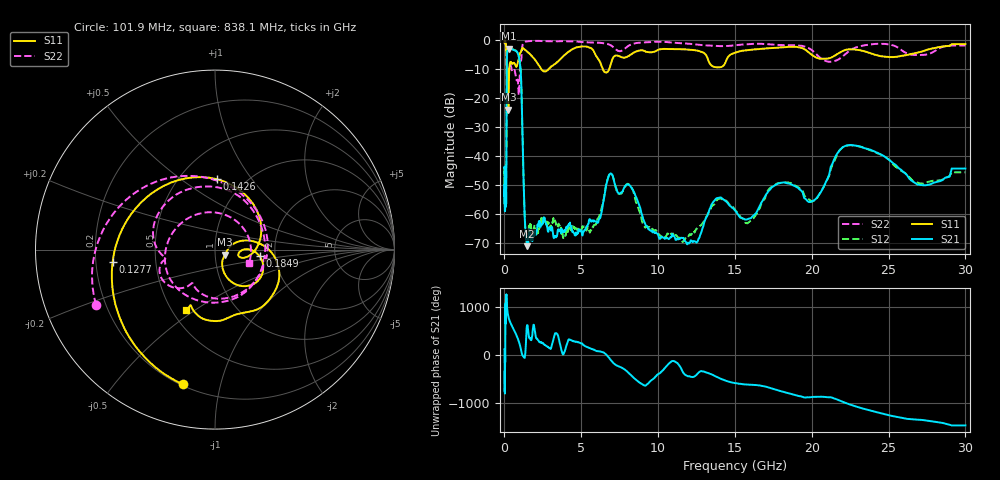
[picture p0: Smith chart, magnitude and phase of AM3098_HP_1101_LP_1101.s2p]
! Date/Time: Thu, Feb 28, 2019 8:46 AM
! Network Analyzer: Agilent Technologies E8364B Rev: A.07.50.67
! Sweep from 0.010 to 30.000 GHz, 1601 Points, Sweep Type: LOG
! Power Supply: 5.022 V, 0.002 A
# Hz S DB R 50
!freq MagS11 AngS11 MagS21 AngS21 MagS12 AngS12 MagS22 AngS22
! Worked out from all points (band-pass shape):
!   1601 points, 10 MHz to 30 GHz, reference 50 ohm
!   highest |S21| = -3.12 dB at 266.5 MHz (marker M1); lowest = -71.2 dB at 1.475 GHz (marker M2)
!   |S21| within 3 dB of the highest: 159.3 MHz to 944.9 MHz (785.6 MHz wide, 142 % of centre)
!   lowest |S11| = -24.1 dB at 252.2 MHz (marker M3), VSWR 1.13, Z = 55.8 - j3.15 ohm
!   |S11| at or under -10 dB: 148 MHz to 316 MHz (168 MHz wide, 72.4 % of centre); 2.372 GHz to 2.902 GHz (529.7 MHz wide, 20.1 % of centre); 6.381 GHz to 6.833 GHz (452.4 MHz wide, 6.85 % of centre)
!   |S22| runs from -19.1 to -0.4 dB; largest |S21 - S12| = 0.012
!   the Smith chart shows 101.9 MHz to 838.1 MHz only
!   S11 on the Smith chart (normalised r, x): 101.9 MHz: 0.21, -0.77; 127.7 MHz: 0.27, -0.06; 142.6 MHz: 0.75, +0.69; 184.9 MHz: 1.65, -0.13; 838.1 MHz: 0.59, -0.46
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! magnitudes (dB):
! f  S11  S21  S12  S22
! 10 MHz  -0.3  -44.3  -44.4  -0.6
! 38.04 MHz  -0.3  -58.3  -58.8  -0.9
! 101.9 MHz  -2.3  -55.3  -56.4  -2.7
! 127.7 MHz  -4.8  -41.3  -41.2  -6.2
! 142.6 MHz  -8.1  -16.8  -16.8  -10.7
! 144.7 MHz  -8.8  -14.3  -14.3  -10.9
! 184.9 MHz  -12.0  -4.1  -4.1  -10.4
! 252.2 MHz  -24.1  -3.2  -3.1  -11.0
! 266.5 MHz  -19.8  -3.1  -3.1  -10.9
! 550.5 MHz  -8.2  -3.5  -3.4  -10.8
! 838.1 MHz  -8.5  -4.4  -4.4  -13.8
! 1.066 GHz  -4.3  -11.4  -11.4  -7.9
! 1.321 GHz  -3.5  -61.6  -61.9  -0.8
! 1.475 GHz  -4.1  -71.2  -69.3  -0.6
! 2.084 GHz  -7.6  -66.5  -66.3  -0.5
! 5.528 GHz  -2.7  -61.9  -66.0  -1.0
! 7.926 GHz  -6.1  -50.1  -50.0  -2.7
! 12.19 GHz  -3.6  -69.4  -67.0  -1.5
! 13.88 GHz  -9.6  -54.6  -55.1  -2.2
! 20.2 GHz  -5.9  -55.2  -55.3  -4.6
! 22.56 GHz  -3.4  -36.3  -36.4  -3.5
! 30 GHz  -1.6  -44.4  -45.8  -2.0
